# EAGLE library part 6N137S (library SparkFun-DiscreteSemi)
Lite-On 6N137 - High Speed Opto Isolator Opto isolator capable of data rates up to 10MBd
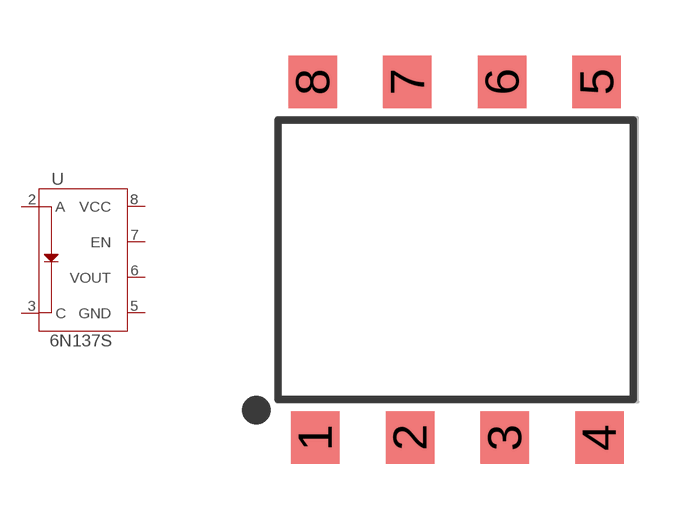
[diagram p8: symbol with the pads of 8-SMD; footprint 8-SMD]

Designator prefix U

## 6N137S (PROD_ID: IC-14151)  [8-SMD]
2  A
3  C
5  GND
6  VOUT
7  EN
8  VCC

## Footprint 8-SMD (pad centres in mm)
smd 1.3 x 1.4: 1 -3.96,-4.96; 2 -1.42,-4.96; 3 1.12,-4.96; 4 3.66,-4.96; 5 3.59,4.58; 6 1.05,4.58; 7 -1.49,4.58; 8 -4.03,4.58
